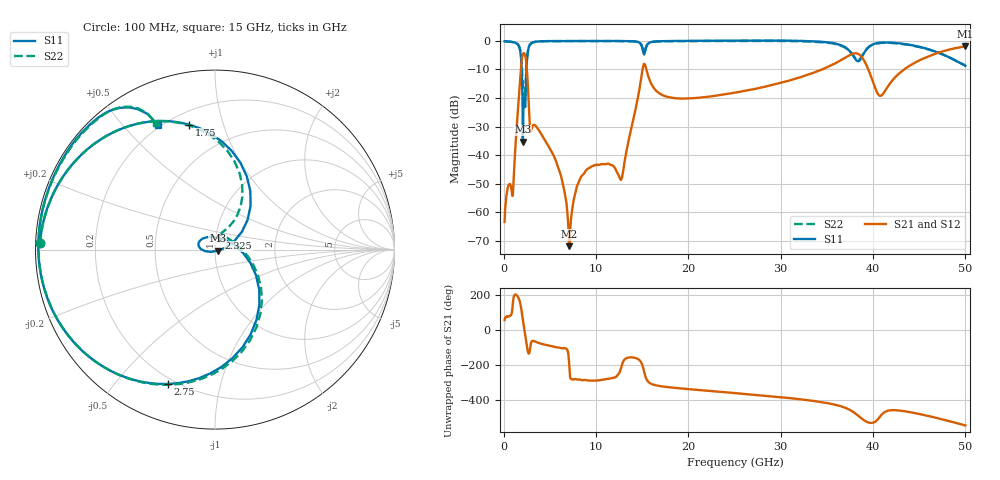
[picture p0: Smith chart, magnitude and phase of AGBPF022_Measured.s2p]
! AWR Design Environment (17559) Fri Feb 23 15:56:34 2024
! Document = 'M073_Measured.AP'
! nPorts: 2, nXvals: 647
# GHz S MA R 50
!Freq MagS11 AngS11 MagS21 AngS21 MagS12 AngS12 MagS22 AngS22
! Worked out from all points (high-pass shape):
!   647 points, 100 MHz to 50 GHz, reference 50 ohm
!   highest |S21| = -2.01 dB at 50 GHz (marker M1); lowest = -71.8 dB at 7.1 GHz (marker M2)
!   |S21| within 3 dB of the highest: 37.49 GHz to 38.57 GHz (1.079 GHz wide, 2.84 % of centre); 46.38 GHz to end of sweep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
!   lowest |S11| = -35.3 dB at 2.075 GHz (marker M3), VSWR 1.04, Z = 51.6 - j0.696 ohm
!   |S11| at or under -10 dB: 1.949 GHz to 2.469 GHz (519.9 MHz wide, 23.5 % of centre)
!   |S22| runs from -20.8 to -0.1 dB; largest |S21 - S12| = 0.0012
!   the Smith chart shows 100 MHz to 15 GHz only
!   S11 on the Smith chart (normalised r, x): 100 MHz: 0.01, +0.02; 1.75 GHz: 0.28, +0.78; 2.325 GHz: 1.04, +0.14; 2.75 GHz: 0.17, -0.69; 15 GHz: 0.19, +0.63
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0.1  0.9759 178.0  0.0006796 57.8  0.0007487 61.7  0.9756 178.0
0.5  0.9677 169.7  0.002923 78.9  0.00289 79.7  0.967 169.7
1  0.9448 156.7  0.002119 157.5  0.002106 157.8  0.9443 156.7
1.75  0.7107 101.6  0.1815 163.5  0.1815 163.5  0.733 105.6
2.075  0.01724 -23.0  0.5799 60.6  0.5798 60.6  0.1505 58.5
2.325  0.06934 70.9  0.5552 -27.2  0.5551 -27.2  0.1303 9.4
2.525  0.4548 -59.4  0.2965 -98.8  0.2964 -98.8  0.491 -61.9
2.75  0.7936 -109.4  0.05863 -133.5  0.05858 -133.6  0.7959 -108.8
3.675  0.9686 -160.9  0.02939 -71.0  0.02939 -71.0  0.9672 -160.8
5.9  0.9857 173.4  0.006054 -99.4  0.006083 -99.6  0.9853 172.7
7.1  0.9863 165.9  0.0002565 160.7  0.0002341 156.5  0.9857 164.9
8.5  0.9864 158.5  0.004405 72.6  0.004384 72.9  0.9848 157.3
12.7  0.9866 138.0  0.003683 141.1  0.003666 140.9  0.9813 136.6
15  0.7606 114.6  0.2878 161.9  0.2878 162.0  0.7775 115.0
16.8  0.9777 127.6  0.1221 40.1  0.1221 40.1  0.9713 125.1
25.1  1.004 90.6  0.1241 -1.6  0.1241 -1.5  0.9872 87.6
33.4  0.9772 51.7  0.27 -45.4  0.2699 -45.4  0.9603 46.1
38.7  0.4907 54.3  0.536 -144.8  0.5359 -144.7  0.5091 43.9
40.6  0.9208 38.6  0.1128 -146.8  0.1128 -146.8  0.9003 27.1
41.7  0.9266 25.5  0.167 -101.6  0.167 -101.5  0.9194 13.1
46.2  0.694 -24.8  0.5479 -135.5  0.5477 -135.4  0.6891 -41.1
50  0.3629 -81.0  0.7936 172.7  0.7933 172.7  0.3701 -103.2
